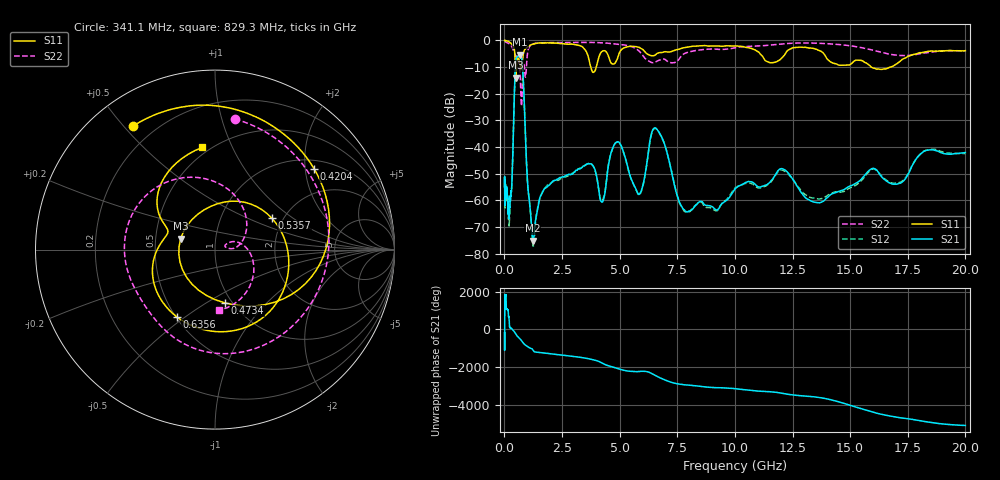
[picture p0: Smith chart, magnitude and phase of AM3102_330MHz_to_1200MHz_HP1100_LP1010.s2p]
! Date/Time: Tue, Sep 11, 2018 5:21 PM
! Network Analyzer: Agilent Technologies E8362B Rev: A.07.50.63
! Sweep from 0.010 to 20.000 GHz, 1601 Points, Sweep Type: LOG
! Power Supply: 4.949 V, 0.001 A
# Hz S DB R 50
!freq MagS11 AngS11 MagS21 AngS21 MagS12 AngS12 MagS22 AngS22
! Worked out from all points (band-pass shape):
!   1601 points, 10 MHz to 20 GHz, reference 50 ohm
!   highest |S21| = -5.34 dB at 685.8 MHz (marker M1); lowest = -75.1 dB at 1.236 GHz (marker M2)
!   |S21| within 3 dB of the highest: 487.9 MHz to 771.9 MHz (283.9 MHz wide, 45.1 % of centre)
!   lowest |S11| = -14.0 dB at 496.5 MHz (marker M3), VSWR 1.50, Z = 33.7 + j4.22 ohm
!   |S11| at or under -10 dB: 696.3 MHz to 754.1 MHz (57.8 MHz wide, 7.97 % of centre); 3.747 GHz to 3.986 GHz (238.7 MHz wide, 6.17 % of centre); 15.91 GHz to 16.76 GHz (847.4 MHz wide, 5.19 % of centre)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
!   |S22| runs from -24.7 to -0.2 dB; largest |S21 - S12| = 0.0093
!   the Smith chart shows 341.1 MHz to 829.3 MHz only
!   S11 on the Smith chart (normalised r, x): 341.1 MHz: 0.12, +0.53; 420.4 MHz: 1.22, +2.23; 473.4 MHz: 0.93, -0.61; 535.7 MHz: 1.74, +0.70; 635.6 MHz: 0.50, -0.46; 829.3 MHz: 0.46, +0.77
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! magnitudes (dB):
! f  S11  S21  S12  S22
! 10 MHz  0.0  -52.5  -55.0  -0.2
! 35.55 MHz  -0.1  -61.4  -60.4  -0.4
! 126.4 MHz  -0.3  -57.7  -59.1  -0.9
! 210.1 MHz  -0.7  -66.4  -68.8  -1.3
! 341.1 MHz  -1.7  -50.0  -50.5  -2.7
! 420.4 MHz  -2.9  -24.1  -24.1  -4.3
! 447.2 MHz  -4.6  -16.2  -16.3  -4.6
! 473.4 MHz  -10.4  -10.4  -10.4  -5.4
! 496.5 MHz  -14.0  -7.6  -7.6  -6.0
! 535.7 MHz  -8.8  -6.4  -6.5  -6.0
! 635.6 MHz  -7.3  -5.5  -5.6  -8.2
! 685.8 MHz  -9.4  -5.3  -5.4  -13.2
! 829.3 MHz  -4.8  -16.4  -16.6  -9.4
! 1.236 GHz  -1.5  -75.1  -77.0  -1.4
! 1.59 GHz  -1.0  -58.1  -58.2  -0.9
! 3.668 GHz  -7.2  -46.3  -46.1  -0.8
! 4.251 GHz  -4.1  -60.7  -60.1  -0.9
! 4.902 GHz  -6.9  -38.1  -38.1  -1.5
! 5.652 GHz  -2.3  -54.9  -55.0  -2.9
! 6.58 GHz  -5.2  -33.0  -33.2  -8.0
! 7.92 GHz  -2.5  -64.4  -64.6  -4.6
! 20 GHz  -3.9  -42.1  -42.5  -3.9
